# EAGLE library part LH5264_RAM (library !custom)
LH5264 RAM Memory used in DMG-01 Original spec sheet cannot be found. This part is based off a currently used SHARP 28SOP footprint (SOP025-P-0450). When compared to scaled photo of DMG pads, this footprint's center of tolerance matches perfectly. Pads extended to 2mm.
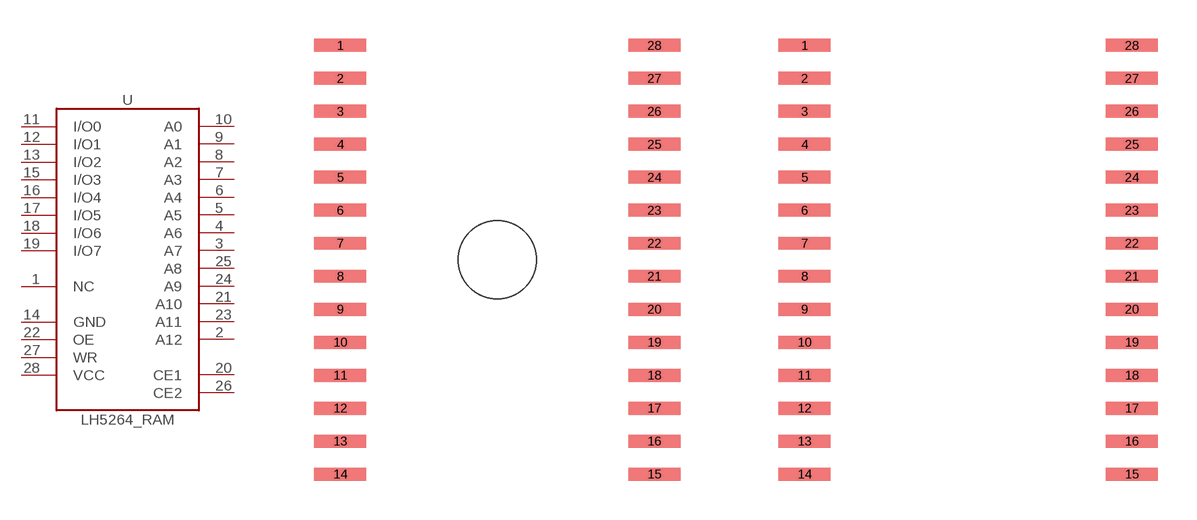
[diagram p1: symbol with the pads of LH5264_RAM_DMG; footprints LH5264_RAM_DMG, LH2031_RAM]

Designator prefix -

## LH5264_RAM_DMG  [LH5264_RAM_DMG]
1  NC  pas
2  A12  pas
3  A7  pas
4  A6  pas
5  A5  pas
6  A4  pas
7  A3  pas
8  A2  pas
9  A1  pas
10  A0  pas
11  I/O0  pas
12  I/O1  pas
13  I/O2  pas
14  GND  pas
15  I/O3  pas
16  I/O4  pas
17  I/O5  pas
18  I/O6  pas
19  I/O7  pas
20  CE1  pas
21  A10  pas
22  OE  pas
23  A11  pas
24  A9  pas
25  A8  pas
26  CE2  pas
27  WR  pas
28  VCC  pas

## LH5264_RAM  [LH2031_RAM]
Pads as for LH5264_RAM_DMG

## Footprint LH5264_RAM_DMG (pad centres in mm)
smd 2 x 0.5: 1 -6.046,8.255; 2 -6.046,6.985; 3 -6.046,5.715; 4 -6.046,4.445; 5 -6.046,3.175; 6 -6.046,1.905; 7 -6.046,0.635; 8 -6.046,-0.635; 9 -6.046,-1.905; 10 -6.046,-3.175; 11 -6.046,-4.445; 12 -6.046,-5.715; 13 -6.046,-6.985; 14 -6.046,-8.255; 15 6.046,-8.255; 16 6.046,-6.985; 17 6.046,-5.715; 18 6.046,-4.445; 19 6.046,-3.175; 20 6.046,-1.905; 21 6.046,-0.635; 22 6.046,0.635; 23 6.046,1.905; 24 6.046,3.175; 25 6.046,4.445; 26 6.046,5.715; 27 6.046,6.985; 28 6.046,8.255
hole 3 at 0,0

## Footprint LH2031_RAM (pad centres in mm)
smd 2 x 0.5: 1 -6.3,8.255; 2 -6.3,6.985; 3 -6.3,5.715; 4 -6.3,4.445; 5 -6.3,3.175; 6 -6.3,1.905; 7 -6.3,0.635; 8 -6.3,-0.635; 9 -6.3,-1.905; 10 -6.3,-3.175; 11 -6.3,-4.445; 12 -6.3,-5.715; 13 -6.3,-6.985; 14 -6.3,-8.255; 15 6.3,-8.255; 16 6.3,-6.985; 17 6.3,-5.715; 18 6.3,-4.445; 19 6.3,-3.175; 20 6.3,-1.905; 21 6.3,-0.635; 22 6.3,0.635; 23 6.3,1.905; 24 6.3,3.175; 25 6.3,4.445; 26 6.3,5.715; 27 6.3,6.985; 28 6.3,8.255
